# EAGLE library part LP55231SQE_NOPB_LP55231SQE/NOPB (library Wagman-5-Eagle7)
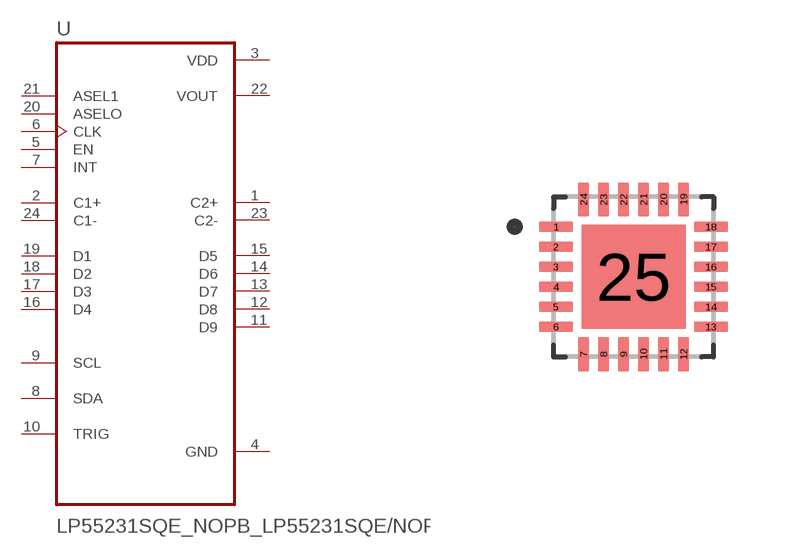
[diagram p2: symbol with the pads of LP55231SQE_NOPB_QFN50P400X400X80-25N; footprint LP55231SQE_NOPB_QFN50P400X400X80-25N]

Designator prefix U

## LP55231SQE_NOPB_LP55231SQE/NOPB (DESCRIPTION: 9 channel RGB / White LED driver with internal program memory and integrated charge Pump - WQFN 24-WQFN -30 to 85; DIGI-KEY_PART_NUMBER: 296-39059-1-ND; MF: Texas Instruments; MP: LP55231SQE/NOPB; PACKAGE: WQFN-24 Texas Instruments; PURCHASE-URL: https://pricing.snapeda.com/search/part/LP55231SQE/NOPB/?ref=eda)  [LP55231SQE_NOPB_QFN50P400X400X80-25N]
1  C2+
2  C1+
3  VDD  pwr
4  GND  pwr
5  EN  in
6  CLK  in
7  INT  in
8  SDA
9  SCL
10  TRIG
11  D9
12  D8
13  D7
14  D6
15  D5
16  D4
17  D3
18  D2
19  D1
20  ASELO  in
21  ASEL1  in
22  VOUT  out
23  C2-
24  C1-

## Footprint LP55231SQE_NOPB_QFN50P400X400X80-25N (pad centres in mm)
smd 0.86 x 0.27: 1 -1.935,1.25; 2 -1.935,0.75; 3 -1.935,0.25; 4 -1.935,-0.25; 5 -1.935,-0.75; 6 -1.935,-1.25; 13 1.935,-1.25; 14 1.935,-0.75; 15 1.935,-0.25; 16 1.935,0.25; 17 1.935,0.75; 18 1.935,1.25
smd 0.27 x 0.86: 7 -1.25,-1.935; 8 -0.75,-1.935; 9 -0.25,-1.935; 10 0.25,-1.935; 11 0.75,-1.935; 12 1.25,-1.935; 19 1.25,1.935; 20 0.75,1.935; 21 0.25,1.935; 22 -0.25,1.935; 23 -0.75,1.935; 24 -1.25,1.935
smd 2.6 x 2.6: 25 0,0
